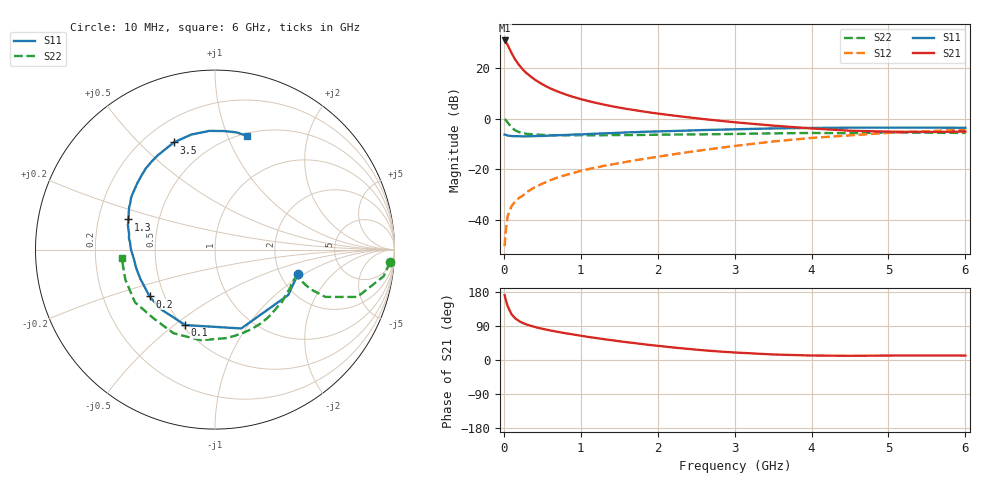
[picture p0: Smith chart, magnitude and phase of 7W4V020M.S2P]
! Infineon Technologies  Discrete & RF Semiconductors
! BFS17W
! Si NPN RF Bipolar Junction Transistor in SOT323
! VCE = 4 V  IC = 20 mA
! Common Emitter S-Parameters:  August  1999
# GHz  S  MA  R  50
!  f  S11  S21  S12  S22
! GHz  MAG  ANG  MAG  ANG  MAG  ANG  MAG  ANG
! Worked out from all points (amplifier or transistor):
!   36 points, 10 MHz to 6 GHz, reference 50 ohm
!   highest |S21| = 30.9 dB at 10 MHz (marker M1)
!   |S21| within 3 dB of that: start of sweep to 68.71 MHz
!   unconditionally stable (mu >= 1): 262.8 MHz to 2.232 GHz; 5.032 GHz to end of sweep
!   at 250 MHz: K = 0.99, MSG = 24.9 dB, |S12| = -30.4 dB
!   at 1.4 GHz: K = 1.17, MAG = 9.0 dB, |S12| = -18.2 dB
!   at 6 GHz: K = 1.06, MAG = -1.8 dB, |S12| = -4.4 dB
!   S11 on the Smith chart (normalised r, x): 10 MHz: 2.50, -0.88; 100 MHz: 0.52, -0.55; 200 MHz: 0.41, -0.27; 1.3 GHz: 0.33, +0.15; 3.5 GHz: 0.32, +0.64; 6 GHz: 0.52, +1.17
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0.01  0.4823 -16.3  35.14 171.4  0.003 88.4  0.9773 -4.1
0.02  0.48 -31.9  34.06 162.7  0.0052 83.2  0.9513 -9.0
0.05  0.463 -71.6  28.51 141.7  0.0119 67.3  0.8355 -18.4
0.1  0.452 -111.5  19.8 120.9  0.0185 59.8  0.6692 -23.2
0.15  0.449 -132.6  14.54 109.4  0.0232 57.9  0.5825 -22.6
0.2  0.4483 -144.4  11.37 102.5  0.0272 61.4  0.5392 -21.2
0.25  0.4439 -152.8  9.261 97.3  0.0303 61.9  0.5138 -19.9
0.3  0.4467 -158.6  7.802 93.4  0.0354 63.6  0.5001 -19.2
0.4  0.4512 -167.1  5.932 87.2  0.0438 66.3  0.4828 -18.7
0.5  0.4541 -172.7  4.774 82.4  0.0516 68.1  0.4772 -19.0
0.6  0.4614 -177.0  3.984 78.1  0.0601 68.7  0.4726 -19.9
0.7  0.4695 179.2  3.438 74.3  0.0686 69.6  0.4701 -21.3
0.9  0.4838 172.4  2.691 67.4  0.0837 70.6  0.4671 -24.9
1.1  0.4961 166.6  2.221 60.8  0.1005 70.8  0.4688 -29.2
1.3  0.511 160.8  1.894 55.0  0.116 71.1  0.4691 -34.1
1.6  0.5342 153.5  1.552 46.9  0.14 71.8  0.4718 -41.7
2.2  0.5693 139.5  1.152 33.1  0.1963 72.0  0.4839 -58.8
2.8  0.604 125.9  0.909 22.4  0.2629 69.3  0.4927 -77.0
3.5  0.6398 111.0  0.727 14.6  0.3528 63.2  0.511 -98.9
4.5  0.6621 92.8  0.576 11.1  0.4665 50.3  0.514 -132.2
5.5  0.664 79.6  0.544 11.9  0.5642 37.3  0.5266 -161.6
6  0.6583 74.5  0.554 11.7  0.6025 31.1  0.5218 -174.7
